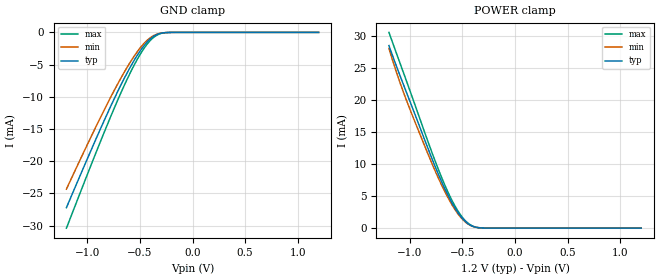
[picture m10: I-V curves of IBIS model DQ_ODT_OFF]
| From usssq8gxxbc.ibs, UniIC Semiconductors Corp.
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|   Model DQ_RCV
[Model] DQ_ODT_OFF
Model_type Input
Polarity   Non-Inverting
Enable   Active-High
Vinl =  8.300E-01
Vinh =  9.700E-01
C_comp   7.319E-13   7.254E-13   7.385E-13
C_comp_power_clamp   3.404E-13   3.388E-13   3.419E-13
C_comp_gnd_clamp   3.758E-13   3.710E-13   3.810E-13
[Model Spec]
Vinh   9.700E-01   9.250E-01   1.015E+00
Vinl   8.300E-01   7.850E-01   8.750E-01
[Temperature Range]   4.500E+01   9.500E+01   0.000E+00
[Voltage Range]   1.200E+00   1.140E+00   1.260E+00
[C Comp Corner]
C_comp_power_clamp   3.404E-13   3.388E-13   3.419E-13
C_comp_gnd_clamp   3.758E-13   3.710E-13   3.810E-13
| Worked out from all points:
|   GND clamp passes 1 mA (typ) near -0.40 V on its own axis
|   POWER clamp passes 1 mA (typ) near -0.47 V on its own axis
[GND_clamp]
|Voltage   I(typ)   I(min)   I(max)
-1.2V     -27.2mA    -24.33mA   -30.38mA
-875mV    -14.93mA   -13.17mA   -16.89mA
-750mV    -10.47mA   -9.157mA   -11.95mA
-650mV    -7.145mA   -6.184mA   -8.244mA
-575mV    -4.884mA   -4.175mA   -5.699mA
-500mV    -2.92mA    -2.45mA    -3.459mA
-425mV    -1.383mA   -1.13mA    -1.679mA
-375mV    -673.2uA   -542.8uA   -837uA
-300mV    -135.5uA   -116.3uA   -166.1uA
-225mV    -14.67uA   -15.93uA   -14.24uA
1.2V      0A         0A         0A
[POWER_clamp]
|Voltage   I(typ)   I(min)   I(max)
-1.2V     28.45mA    28mA       30.5mA
-1.125V   25.07mA    24.12mA    27.08mA
-1.025V   20.8mA     19.57mA    22.55mA
-850mV    13.34mA    12.42mA    14.46mA
-750mV    9.2mA      8.545mA    10.01mA
-650mV    5.523mA    5.115mA    6.037mA
-575mV    3.235mA    2.981mA    3.547mA
-500mV    1.501mA    1.371mA    1.657mA
-450mV    723.1uA    662.7uA    804.4uA
-375mV    148.3uA    148.7uA    156.1uA
-300mV    17.6uA     22.56uA    14.19uA
1.2V      0A         0A         0A
